FUNCTION F_Crc6 : BYTE
VAR_INPUT
END_VAR
VAR_IN_OUT
	aData			: ARRAY[*] OF USINT;
END_VAR
VAR
	nLowBoundData	: DINT;			// lower index
	nUpBoundData	: DINT;			// upper index
	nIdxCntData		: DINT;			// number elements  
	
	aCrc6Table 		: ARRAY[0..63] OF BYTE:=[	0, 25, 50, 43, 61, 36, 15, 22, 35, 58, 17, 8, 30, 7, 44, 53,
												31, 6, 45, 52, 34, 59, 16, 9, 60, 37, 14, 23, 1, 24, 51, 42,
												62, 39, 12, 21, 3, 26, 49, 40, 29, 4, 47, 54, 32, 57, 18, 11,
												33, 56, 19, 10, 28, 5, 46, 55, 2, 27, 48, 41, 63, 38, 13, 20 ];		// CRC lookup table
	nIdx			: DINT;
	nRetBuff		: BYTE;
END_VAR

// check if input array is not there
IF aData <> 0 THEN
	// get array dimensions 
	nLowBoundData := LOWER_BOUND(aData, 1);
	nUpBoundData := UPPER_BOUND(aData, 1);
	IF nLowBoundData = nUpBoundData THEN
		nIdxCntData := 1;
	ELSE
		nIdxCntData := nUpBoundData - nLowBoundData + 1;	
	END_IF


	nRetBuff:=21;
	
	FOR nIdx := nLowBoundData TO nUpBoundData DO
		nRetBuff := aData[nIdx] XOR aCrc6Table[nRetBuff + 1];
	END_FOR
	
	nRetBuff := 0 XOR aCrc6Table[nRetBuff + 1];

END_IF

 F_Crc6 := nRetBuff;

END_FUNCTION
